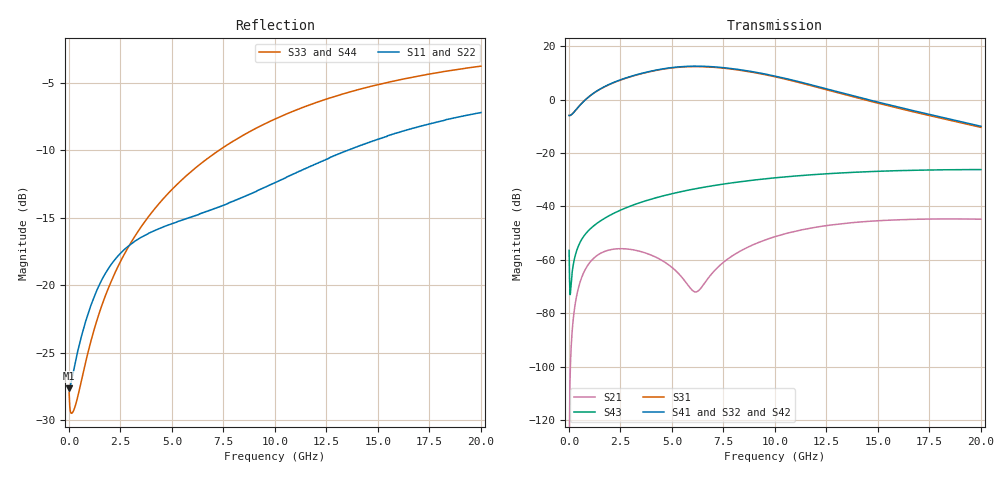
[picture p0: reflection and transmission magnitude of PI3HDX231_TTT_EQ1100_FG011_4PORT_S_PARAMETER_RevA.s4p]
! NPort=4 DATA=2000 NOISE=0 GROUPDELAY=0 COMPLEX_DATAFORMAT=POLAR
! NumOfBlock=1 NumOfParam=0
! .MODEL Smodel S TSTONEFILE=PI3HDX231_TTT_EQ1100_FG011_4PORT_S_PARAMETER_RevA.s4p TYPE=S
!  -- The above .MODEL line can be used for the S element in the netlist.
! The s parameter is extracted from the linear redriver, it is not bi-directional; only s(4,1)s(4,2) and s(3,1)s(3,2)
! should be the insertion loss
!Port definition:
!Port1 = input+
!Port2 = input-
!Port3 = output+
!Port4 = output-
# Hz S MA R  50
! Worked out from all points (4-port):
!   2000 points, 10 MHz to 20 GHz, reference 50 ohm
!   strongest paths, dB at 10 MHz, 5.01 GHz, 10.01 GHz, 15.01 GHz, 20 GHz:
!     S41: -5.9, 12.0, 8.8, -1.0, -10.0
!     S32: -5.9, 11.9, 8.7, -1.0, -9.9
!     S42: -5.9, 12.0, 8.7, -1.1, -10.1
!     S31: -5.9, 11.9, 8.5, -1.4, -10.4
!     S43: -56.5, -35.2, -29.3, -26.8, -26.2
!     S21: -134.8, -62.9, -51.3, -45.4, -44.8
!   lowest |S11| = -27.6 dB at 10 MHz (marker M1), VSWR 1.09, Z = 46 - j0.0776 ohm
!   |S11| at or under -10 dB: start of sweep to 13.55 GHz
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1e7  0.04152 -178.8  1.825e-07 -14.0  0 0.0  0 0.0
     1.825e-07 -13.9  0.04152 -178.8  0 0.0  0 0.0
     0.5043 0.3  0.5043 -179.7  0.04012 -3.2  0.0015 -70.3
     0.5043 -179.7  0.5043 0.3  0.0015 -70.3  0.04012 -3.2
3.81e9  0.1548 -141.0  0.001305 -0.3  1.409e-10 -138.3  1.083e-10 -127.3
        0.001305 -0.2  0.1548 -141.1  1.031e-10 -128.0  1.476e-10 -137.4
        3.254 -38.8  3.262 141.0  0.1771 -98.6  0.01305 67.6
        3.296 141.2  3.286 -38.0  0.01303 67.5  0.1771 -98.6
5.77e9  0.1772 -138.7  0.000337 4.0  1.674e-09 159.4  1.101e-09 -174.0
        0.0003401 4.7  0.177 -138.9  1.039e-09 -173.0  1.769e-09 159.3
        4.128 -101.1  4.147 78.7  0.2572 -104.7  0.02012 57.2
        4.197 78.7  4.183 -100.2  0.02006 57.1  0.2573 -104.7
7.85e9  0.2031 -133.8  0.00113 101.8  9.607e-09 96.0  6.895e-09 131.9
        0.00113 101.2  0.2025 -134.0  6.601e-09 134.2  1.012e-08 94.7
        3.747 -167.7  3.788 12.1  0.3364 -110.3  0.02749 44.5
        3.832 11.8  3.807 -166.8  0.02739 44.6  0.3366 -110.3
1.05e10  0.2493 -129.0  0.003088 79.9  4.123e-08 22.9  3.266e-08 56.3
         0.003082 79.6  0.2479 -129.2  3.197e-08 59.1  4.275e-08 20.7
         2.42 117.8  2.477 -62.6  0.428 -116.8  0.03581 27.3
         2.497 -63.2  2.466 118.9  0.03571 27.5  0.428 -116.9
1.35e10  0.3148 -128.4  0.004876 48.5  1.156e-07 -46.5  9.241e-08 -20.3
         0.004859 48.3  0.3128 -128.4  9.219e-08 -17.6  1.177e-07 -48.9
         1.208 52.2  1.258 -129.2  0.5151 -123.5  0.04297 7.7
         1.261 -129.9  1.237 53.4  0.04293 8.0  0.515 -123.5
2e10  0.4356 -135.6  0.005795 -4.0  3.838e-07 -162.4  2.874e-07 -145.3
      0.005765 -4.2  0.4339 -135.4  2.918e-07 -143.8  3.827e-07 -164.3
      0.3021 -49.4  0.3194 125.5  0.6464 -135.0  0.04884 -32.3
      0.3172 125.0  0.3128 -48.2  0.04896 -32.1  0.6461 -135.0
